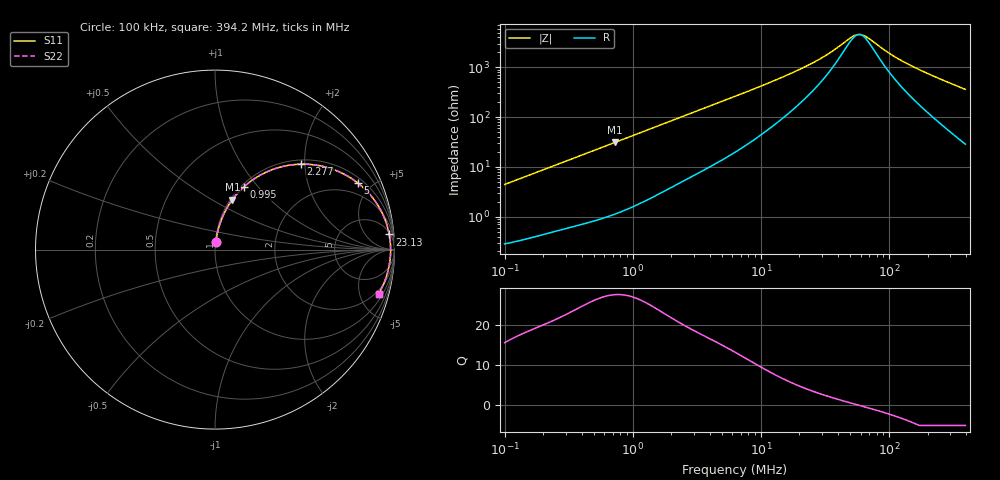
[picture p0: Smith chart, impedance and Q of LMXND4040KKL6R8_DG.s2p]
! LMXND4040KKL6R8_DG  S-PARAMETER MODEL  ( General Type )
! Model Generated by TAIYO YUDEN Corporation (http://www.ty-top.com)
! Version 1.0
! TAIYO YUDEN Control No. 191023NI43SB-FBB
! Copyright(c) 2019 TAIYO YUDEN CO.,LTD. All Rights Reserved.
! Product Description (link to TY-COMPAS)
! https://ds.yuden.co.jp/TYCOMPAS/or/detail?pn=LMXND4040KKL6R8MDG&u=M
! Products Name : Inductors
! Characteristics :
!  Inductance : 6.8 uH , SRF(min) : 38 MHz , DC Resistance(max) : 0.24 Ohm
!  Rated Current : Saturation :800 mA , Temp Rise : 1000 mA
!  Case Size : 4.0 x 4.0 / 0.157 x 0.157 [mm/inch] , Thickness : 1 / 0.039 [mm/inch]
!  (Conditions: Temperature = 25 degC , DC Bias Current/Voltage = 0A / 0V)
! External Node Assignments :
!  1  o---GGG---o  2
! GND o---------o GND
! Frequency Range : 0.1MHz  -  394.189695MHz  [ 402 STEP ]
# MHz S RI R 50
! Freq[MHz].  S11 Real  S11 Imag  S21 Real  S21 Imag  S12 Real  S12 Imag  S22 Real  S22 Imag
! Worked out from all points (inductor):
!   401 points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, 100 kHz to 394.2 MHz, reference 50 ohm
!   read as one part in series: L = 7.02 uH near 104.2 kHz
!   highest Q = 27.5 at 729.4 kHz (marker M1), where L = 6.79 uH
!   self-resonance near 58.45 MHz
!   S11 on the Smith chart (normalised r, x): 100 kHz: 1.01, +0.09; 995 kHz: 1.03, +0.85; 2.277 MHz: 1.09, +1.91; 5 MHz: 1.28, +4.14; 23.13 MHz: 6, +21; 394.2 MHz: 1.57, -7.20
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0.1  0.00477 0.0439  0.9952 -0.0439  0.9952 -0.0439  0.00477 0.0439
0.210675  0.0128 0.0904  0.9872 -0.0904  0.9872 -0.0904  0.0128 0.0904
0.400203  0.0352 0.1651  0.9648 -0.1651  0.9648 -0.1651  0.0352 0.1651
0.729406  0.0968 0.2781  0.9032 -0.2781  0.9032 -0.2781  0.0968 0.2781
0.994966  0.1611 0.3495  0.8389 -0.3495  0.8389 -0.3495  0.1611 0.3495
1.601627  0.3213 0.4463  0.6787 -0.4463  0.6787 -0.4463  0.3213 0.4463
2.277082  0.4788 0.476  0.5212 -0.476  0.5212 -0.476  0.4788 0.476
3.237399  0.6387 0.4535  0.3613 -0.4535  0.3613 -0.4535  0.6387 0.4535
5.000008  0.7963 0.3707  0.2037 -0.3707  0.2037 -0.3707  0.7963 0.3707
6.278453  0.854 0.3173  0.146 -0.3173  0.146 -0.3173  0.854 0.3173
10.979  0.9352 0.1958  0.0648 -0.1958  0.0648 -0.1958  0.9352 0.1958
23.13003  0.9708 0.0847  0.0292 -0.0847  0.0292 -0.0847  0.9708 0.0847
25.12657  0.9724 0.0755  0.0276 -0.0755  0.0276 -0.0755  0.9724 0.0755
34.99141  0.9766 0.0429  0.0234 -0.0429  0.0234 -0.0429  0.9766 0.0429
50.78883  0.9785 0.0113  0.0215 -0.0113  0.0215 -0.0113  0.9785 0.0113
57.50476  0.9786 0.00131  0.0214 -0.00131  0.0214 -0.00131  0.9786 0.00131
61.18875  0.9786 -0.00367  0.0214 0.00367  0.0214 0.00367  0.9786 -0.00367
66.47045  0.9785 -0.0103  0.0215 0.0103  0.0215 0.0103  0.9785 -0.0103
100.5574  0.9766 -0.0456  0.0234 0.0456  0.0234 0.0456  0.9766 -0.0456
128.9095  0.9737 -0.0699  0.0263 0.0699  0.0263 0.0699  0.9737 -0.0699
175.8426  0.9671 -0.106  0.0329 0.106  0.0329 0.106  0.9671 -0.106
394.1897  0.912 -0.2464  0.088 0.2464  0.088 0.2464  0.912 -0.2464
